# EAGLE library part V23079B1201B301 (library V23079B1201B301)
TE CONNECTIVITY / AXICOM - V23079B1201B301 - RELAY, SIGNAL, DPDT, 250VAC, 220VDC, 2A Source: Datasheet
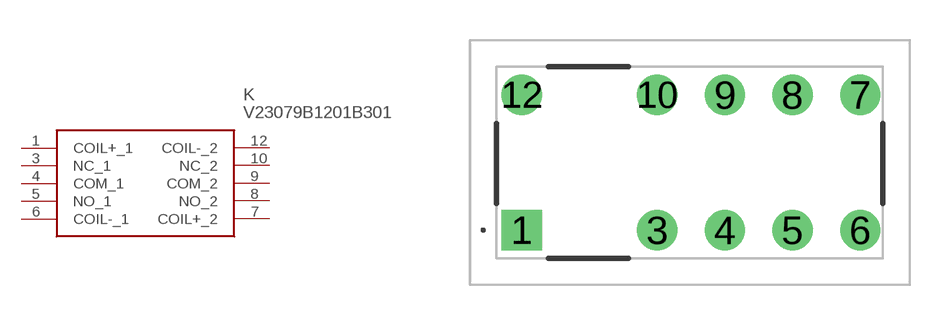
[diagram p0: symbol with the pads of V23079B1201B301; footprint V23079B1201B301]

Designator prefix K

## V23079B1201B301 (Description: TE CONNECTIVITY / AXICOM - V23079B1201B301 - RELAY, SIGNAL, DPDT, 250VAC, 220VDC, 2A; Height: 9.9mm; Manufacturer_Name: TE Connectivity; Manufacturer_Part_Number: V23079B1201B301; Mouser_Part_Number: 655-V23079B1201B301; Mouser_Price-Stock: https://www.mouser.co.uk/ProductDetail/TE-Connectivity-Axicom/V23079B1201B301?qs=Mpp7pS3%252Boa448t%252ByTVqVnw%3D%3D)  [V23079B1201B301]
1  COIL+_1
3  NC_1
4  COM_1
5  NO_1
6  COIL-_1
7  COIL+_2
8  NO_2
9  COM_2
10  NC_2
12  COIL-_2

## Footprint V23079B1201B301 (pad centres in mm)
V23079B1201B301-1
drill 1 pad 1.5 square: 1 0,0
drill 1 pad 1.5: 3 5.08,0; 4 7.62,0; 5 10.16,0; 6 12.7,0; 7 12.7,5.08; 8 10.16,5.08; 9 7.62,5.08; 10 5.08,5.08; 12 0,5.08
